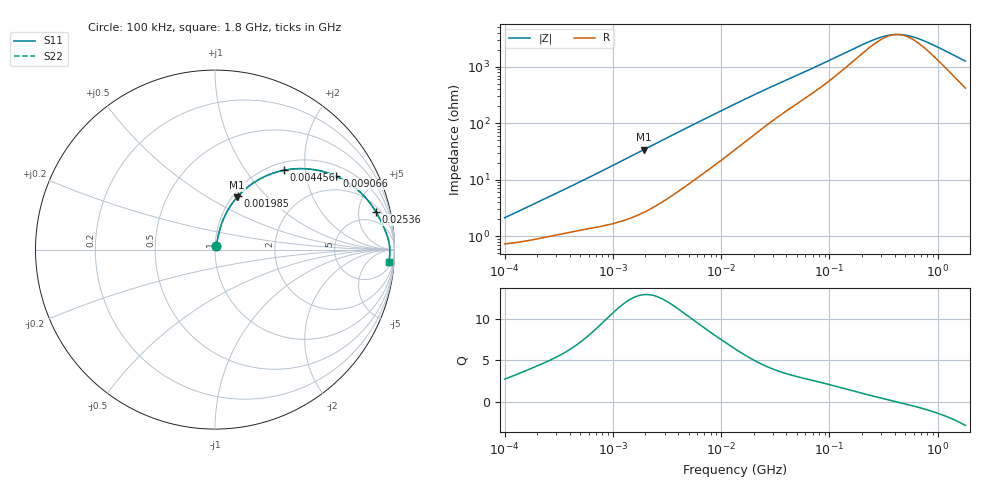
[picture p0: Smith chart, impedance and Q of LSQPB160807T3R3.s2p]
! LSQPB160807T3R3  S-PARAMETER MODEL  ( General Type )
! Model Generated by TAIYO YUDEN Corporation (http://www.ty-top.com)
! Version 1.0
! TAIYO YUDEN Control No. 110308NG25SB-FKC
! Copyright(c) 2011 TAIYO YUDEN CO.,LTD. All Rights Reserved.
! Product Description (link to TY-COMPAS)
! https://ds.yuden.co.jp/TYCOMPAS/or/detail?pn=LSQPB160807T3R3M&u=M
! Products Name : Inductors
! Characteristics :
!  Inductance : 3.3 uH , SRF(min) : 300 MHz , DC Resistance(max) : 0.845 Ohm
!  Rated Current : Saturation :290 mA , Temp Rise : 390 mA (40 degC)
!  Case Size : 1.6 x 0.8 / 0.063 x 0.031 [mm/inch] , Thickness : 0.7 / 0.028 [mm/inch]
!  (Conditions: Temperature = 25 degC , DC Bias Current/Voltage = 0A / 0V)
! External Node Assignments :
!  1  o---GGG---o  2
! GND o---------o GND
! Frequency Range : 0.1MHz  -  1800MHz  [ 402 STEP ]
# MHz S RI R 50
! Freq[MHz].  S11 Real  S11 Imag  S21 Real  S21 Imag  S12 Real  S12 Imag  S22 Real  S22 Imag
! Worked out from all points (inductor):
!   401 points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, 100 kHz to 1.8 GHz, reference 50 ohm
!   read as one part in series: L = 3.13 uH near 115.8 kHz
!   highest Q = 12.9 at 1.937 MHz (marker M1), where L = 2.8 uH
!   self-resonance near 417.9 MHz
!   S11 on the Smith chart (normalised r, x): 100 kHz: 1.01, +0.04; 1.985 MHz: 1.05, +0.70; 4.456 MHz: 1.14, +1.53; 9.066 MHz: 1.38, +3.01; 25.36 MHz: 2.76, +7.65; 1.8 GHz: 9, -24
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0.1  0.00764 0.0196  0.9924 -0.0196  0.9924 -0.0196  0.00764 0.0196
0.253659  0.012 0.0474  0.988 -0.0474  0.988 -0.0474  0.012 0.0474
0.516129  0.0212 0.0911  0.9788 -0.0911  0.9788 -0.0911  0.0212 0.0911
1.130264  0.0544 0.1869  0.9456 -0.1869  0.9456 -0.1869  0.0544 0.1869
1.937403  0.1228 0.2916  0.8772 -0.2916  0.8772 -0.2916  0.1228 0.2916
1.985446  0.1275 0.297  0.8725 -0.297  0.8725 -0.297  0.1275 0.297
2.66389  0.1977 0.3605  0.8023 -0.3605  0.8023 -0.3605  0.1977 0.3605
4.455722  0.3825 0.4416  0.6175 -0.4416  0.6175 -0.4416  0.3825 0.4416
6.278453  0.53 0.4483  0.47 -0.4483  0.47 -0.4483  0.53 0.4483
9.066201  0.6763 0.4085  0.3237 -0.4085  0.3237 -0.4085  0.6763 0.4085
13.41641  0.7935 0.3338  0.2065 -0.3338  0.2065 -0.3338  0.7935 0.3338
18.00091  0.8523 0.2734  0.1477 -0.2734  0.1477 -0.2734  0.8523 0.2734
25.36465  0.8965 0.2105  0.1035 -0.2105  0.1035 -0.2105  0.8965 0.2105
40.39749  0.9313 0.1448  0.0687 -0.1448  0.0687 -0.1448  0.9313 0.1448
69.24595  0.9541 0.0915  0.0459 -0.0915  0.0459 -0.0915  0.9541 0.0915
229.9669  0.9724 0.0218  0.0276 -0.0218  0.0276 -0.0218  0.9724 0.0218
293.7968  0.9733 0.0124  0.0267 -0.0124  0.0267 -0.0124  0.9733 0.0124
357.3983  0.9737 0.00545  0.0263 -0.00545  0.0263 -0.00545  0.9737 0.00545
467.921  0.974 -0.00394  0.026 0.00394  0.026 0.00394  0.974 -0.00394
627.8136  0.9739 -0.0146  0.0261 0.0146  0.0261 0.0146  0.9739 -0.0146
884.6373  0.9734 -0.0286  0.0266 0.0286  0.0266 0.0286  0.9734 -0.0286
1800  0.9691 -0.0707  0.0309 0.0707  0.0309 0.0707  0.9691 -0.0707
